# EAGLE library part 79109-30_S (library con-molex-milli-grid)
RECEPTACAL
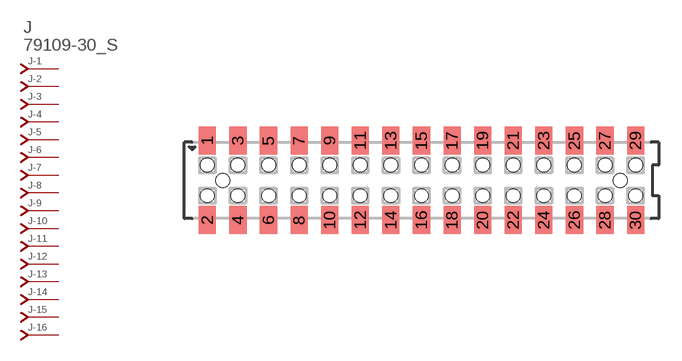
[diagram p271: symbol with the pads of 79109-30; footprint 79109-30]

Designator prefix J; gates -1=J-NV -2=J-N -3=J-N -4=J-N -5=J-N -6=J-N -7=J-N -8=J-N -9=J-N -10=J-N -11=J-N -12=J-N -13=J-N -14=J-N -15=J-N -16=J-N -17=J-N -18=J-N -19=J-N -20=J-N -21=J-N -22=J-N -23=J-N -24=J-N -25=J-N -26=J-N -27=J-N -28=J-N -29=J-N -30=J-N

## 79109-30_S  [79109-30]
1  -1:J  pas
2  -2:J  pas
3  -3:J  pas
4  -4:J  pas
5  -5:J  pas
6  -6:J  pas
7  -7:J  pas
8  -8:J  pas
9  -9:J  pas
10  -10:J  pas
11  -11:J  pas
12  -12:J  pas
13  -13:J  pas
14  -14:J  pas
15  -15:J  pas
16  -16:J  pas
17  -17:J  pas
18  -18:J  pas
19  -19:J  pas
20  -20:J  pas
21  -21:J  pas
22  -22:J  pas
23  -23:J  pas
24  -24:J  pas
25  -25:J  pas
26  -26:J  pas
27  -27:J  pas
28  -28:J  pas
29  -29:J  pas
30  -30:J  pas

## Footprint 79109-30 (pad centres in mm)
RECEPTACAL SMD Dual Row, Vertical, Pass-Thru
smd 1.12 x 1.83: 1 -14,2.6; 2 -14,-2.6; 3 -12,2.6; 4 -12,-2.6; 5 -10,2.6; 6 -10,-2.6; 7 -8,2.6; 8 -8,-2.6; 9 -6,2.6; 10 -6,-2.6; 11 -4,2.6; 12 -4,-2.6; 13 -2,2.6; 14 -2,-2.6; 15 0,2.6; 16 0,-2.6; 17 2,2.6; 18 2,-2.6; 19 4,2.6; 20 4,-2.6; 21 6,2.6; 22 6,-2.6; 23 8,2.6; 24 8,-2.6; 25 10,2.6; 26 10,-2.6; 27 12,2.6; 28 12,-2.6; 29 14,2.6; 30 14,-2.6
hole 0.914 at -13,0
hole 0.914 at -14,1
hole 0.914 at -14,-1
hole 0.914 at -12,-1
hole 0.914 at -12,1
hole 0.914 at -10,-1
hole 0.914 at -10,1
hole 0.914 at 13,0
hole 0.914 at -8,1
hole 0.914 at -8,-1
hole 0.914 at -6,1
hole 0.914 at -6,-1
hole 0.914 at -4,1
hole 0.914 at -4,-1
hole 0.914 at -2,1
hole 0.914 at -2,-1
hole 0.914 at 0,-1
hole 0.914 at 0,1
hole 0.914 at 2,1
hole 0.914 at 2,-1
hole 0.914 at 4,1
hole 0.914 at 4,-1
hole 0.914 at 6,1
hole 0.914 at 6,-1
hole 0.914 at 8,-1
hole 0.914 at 8,1
hole 0.914 at 10,1
hole 0.914 at 12,1
hole 0.914 at 14,1
hole 0.914 at 10,-1
hole 0.914 at 12,-1
hole 0.914 at 14,-1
